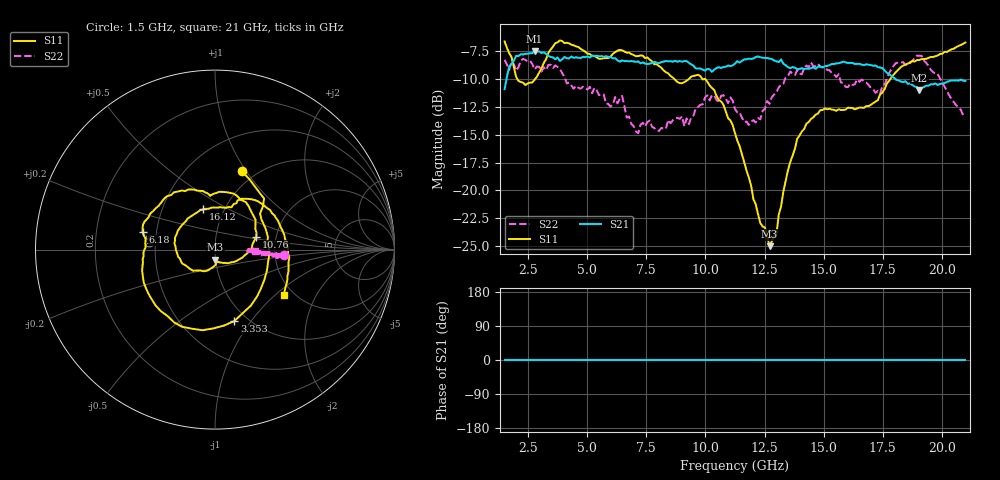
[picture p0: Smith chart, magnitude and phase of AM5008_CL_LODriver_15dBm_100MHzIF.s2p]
!Keysight Technologies,N5245B,MY58422270,A.16.20.02
!Mixer S2P File: Scalar Mixer Measurement
!Calibration State: On
!Parameters: Stimulus Freq, S11, SC21, SC12, S22
# Hz  S  DB  R  50.0
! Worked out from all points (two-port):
!   201 points, 1.5 GHz to 21 GHz, reference 50 ohm
!   highest |S21| = -7.54 dB at 2.768 GHz (marker M1); lowest = -11.0 dB at 19.05 GHz (marker M2)
!   |S21| within 3 dB of the highest: 1.536 GHz to 18.73 GHz (17.19 GHz wide, 170 % of centre); 19.87 GHz to end of sweep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
!   lowest |S11| = -25.0 dB at 12.71 GHz (marker M3), VSWR 1.12, Z = 49.9 - j5.64 ohm
!   |S11| at or under -10 dB: 2.028 GHz to 2.809 GHz (780.9 MHz wide, 32.3 % of centre); 8.659 GHz to 9.318 GHz (659.2 MHz wide, 7.33 % of centre); 9.858 GHz to 17.84 GHz (7.982 GHz wide, 57.6 % of centre)
!   |S22| runs from -14.9 to -8.0 dB; largest |S21 - S12| = 0.42
!   S11 on the Smith chart (normalised r, x): 1.5 GHz: 0.86, +0.96; 3.353 GHz: 0.87, -0.83; 6.18 GHz: 0.42, +0.10; 10.76 GHz: 1.58, +0.24; 16.12 GHz: 0.80, +0.38; 21 GHz: 1.77, -1.13
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1.5e9  -6.69 71.1  -10.95 0.0  -200.00 90.0  -8.34 -4.3
2.085e9  -10.21 33.0  -8.00 0.0  -200.00 90.0  -8.98 -4.9
2.7675e9  -10.12 -21.9  -7.54 0.0  -200.00 90.0  -9.19 -6.0
3.3525e9  -7.69 -75.0  -7.98 0.0  -200.00 90.0  -8.78 -4.1
3.645e9  -6.85 -98.8  -8.28 0.0  -200.00 90.0  -8.83 -5.8
4.1325e9  -6.80 -131.6  -8.19 0.0  -200.00 90.0  -10.43 -3.4
4.815e9  -7.47 -163.5  -8.06 0.0  -200.00 90.0  -10.73 -6.1
6.18e9  -7.64 166.4  -8.18 0.0  -200.00 90.0  -11.66 -1.7
7.0575e9  -8.01 142.1  -8.52 0.0  -200.00 90.0  -14.73 0.7
8.0325e9  -8.89 111.3  -8.63 0.0  -200.00 90.0  -14.68 -4.1
9.69e9  -9.67 71.5  -9.10 0.0  -200.00 90.0  -12.53 -2.9
1.07625e10  -12.35 17.3  -8.97 0.0  -200.00 90.0  -11.49 -4.0
1.125e10  -14.88 -6.8  -8.67 0.0  -200.00 90.0  -12.72 -4.5
1.1835e10  -18.84 -38.5  -8.22 0.0  -200.00 90.0  -14.15 -3.3
1.27125e10  -24.97 -87.9  -8.22 0.0  -200.00 90.0  -12.26 -5.7
1.38825e10  -15.39 -136.3  -9.18 0.0  -200.00 90.0  -9.24 -3.4
1.4565e10  -13.46 -174.7  -9.01 0.0  -200.00 90.0  -8.92 -5.8
1.6125e10  -12.63 106.3  -8.60 0.0  -200.00 90.0  -10.46 -3.9
1.73925e10  -11.43 68.1  -9.01 0.0  -200.00 90.0  -11.37 -5.8
1.77825e10  -10.19 64.0  -9.61 0.0  -200.00 90.0  -9.48 -4.8
1.905e10  -8.35 27.8  -11.02 0.0  -200.00 90.0  -7.97 -4.8
2.1e10  -6.78 -33.4  -10.22 0.0  -200.00 90.0  -13.11 -1.3
